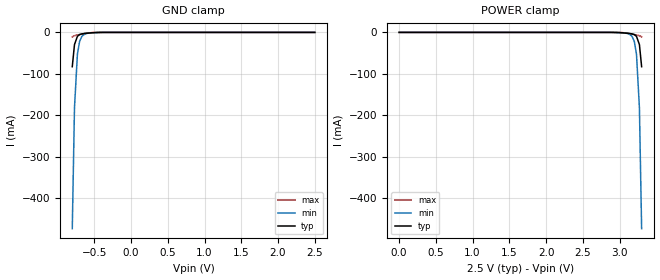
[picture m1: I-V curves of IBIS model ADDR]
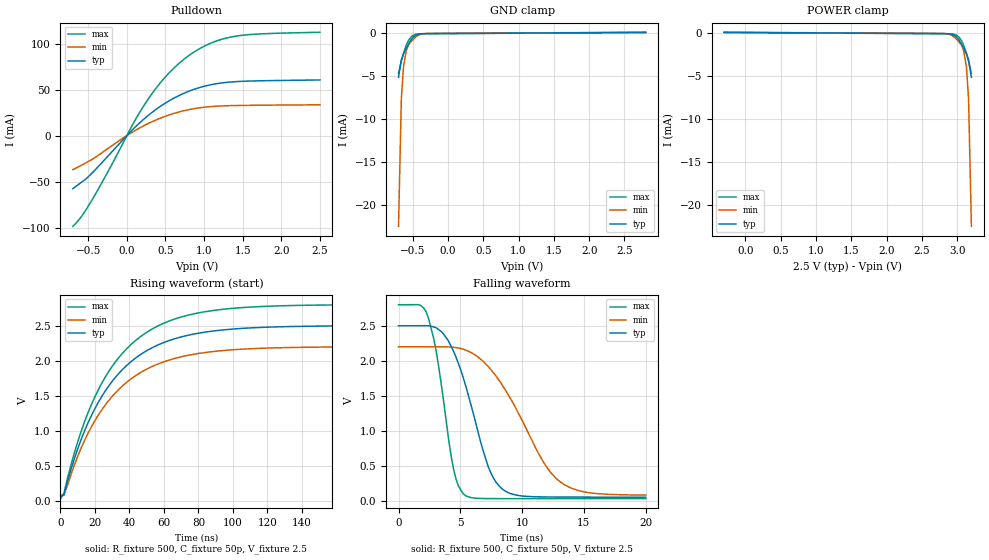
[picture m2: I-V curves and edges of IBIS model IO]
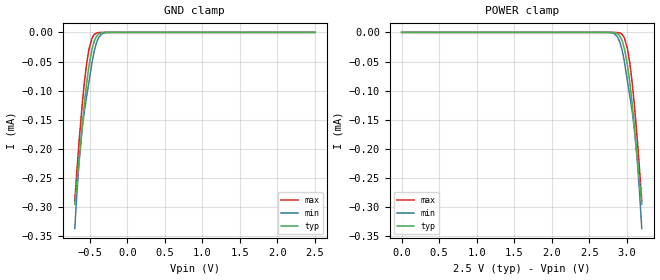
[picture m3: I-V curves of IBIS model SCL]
[IBIS Ver]   3.2
[Comment Char]   |_char
| VDD nom = 2.5v, min = 2.2v, max = 2.8v
[File name]   pca8575_2_5v.ibs
[File Rev]   1
[Date]   Aug 14, 2008 2:49:03 PM
[Source]
Generated by Seshadri Venkataramanan using IBIS Toolkit at NXP Tempe
[Notes]
[Disclaimer]
(C) Copyright 2007 NXP Semiconductors
All rights reserved
NXP Semiconductors (NXP) does not warrant that this model and any other
accompanying information (Model) accurately or fully represents the
operating characteristics and specifications of the semiconductor
products to which the Model relates.  Moreover, the Model is furnished
on an "as is" and with "all faults" basis, and without support or
warranty of any kind.  NXP disclaims all warranties, whether expressed
or implied or statutory, including without limitation all implied
warranties of non-infringement, merchantability and fitness for any
purpose, and those arising from a course of dealing or usage of trade.
NXP does not convey any license under its or any third party's patents,
copyrights or other intellectual property or proprietary rights.
You and your company assume any and all risks and liability arising out
of the application or use of the Model.
In no event shall NXP be liable for any direct, indirect, special,
consequential or incidental damages, however caused, whether in
warranty, contract or tort (including negligence), strict liability or
other legal theory, including, without limitation, for lost profits,
business interruption, or corruption or loss of data or information,
arising out of or in connection with the use of or the inability to use
the Model, even if NXP has been advised of the possibility of such
damages.
NXP provides the Model as a courtesy to our customers. You and your
company shall not distribute, convey, sell, or give the Model to anyone
else without receiving prior written permission from NXP.
NXP reserves the right to make changes without notice to the Model to
improve reliability, function, or design.
Please be aware that your receipt and subsequent use of the Model shall
serve as acceptance of these terms and conditions.  If you do not
accept these terms, return or destroy the Model immediately.
[Copyright]
2008
| SO24 package
[Component]   PCA8575D
Si_location Pin
Timing_location Pin
[Manufacturer]   NXP Semiconductors
[Package]
R_pkg   0.14   0.12   0.18
L_pkg   5.71n   3.95n   7.95n
C_pkg   1.01p   0.72p   1.49p
[Pin] signal_name   model_name   R_pin   L_pin   C_pin
1   INTb   INT_OUT   0.18   6.01n   0.97p
2   AD1   ADDR   0.14   7.94n   1.21p
3   AD2   ADDR   0.16   7.06n   1.32p
4   P00   IO   0.18   6.01n   1.07p
5   P01   IO   0.14   4.98n   0.88p
6   P02   IO   0.13   4.30n   0.80p
7   P03   IO   0.12   3.95n   0.74p
8   P04   IO   0.12   3.95n   0.72p
9   P05   IO   0.13   4.30n   0.76p
10   P06   IO   0.14   4.98n   0.85p
11   P07   IO   0.18   6.01n   0.97p
12   VSS   GND   0.16   7.06n   1.20p
13   P10   IO   0.14   7.95n   1.45p
14   P11   IO   0.14   7.95n   1.49p
15   P12   IO   0.16   7.06n   1.32p
16   P13   IO   0.18   6.01n   1.07p
17   P14   IO   0.14   4.98n   0.88p
18   P15   IO   0.13   4.30n   0.80p
19   P16   IO   0.12   3.95n   0.74p
20   P17   IO   0.12   3.95n   0.72p
21   AD0   ADDR   0.13   4.30n   0.76p
22   SCL   SCL   0.14   4.98n   0.85p
23   SDA   SDAIO   0.18   6.01n   0.97p
24   VDD   POWER   0.16   7.06n   1.20p
| TSSOP24 package
[Component]   PCA8575PW
Si_location Pin
Timing_location Pin
[Manufacturer]   NXP Semiconductors
[Package]
R_pkg   52.70m   31.50m   67.00m
L_pkg   2.19n   1.32n   3.39n
C_pkg   0.48p   0.35p   0.93p
[Pin] signal_name   model_name   R_pin   L_pin   C_pin
1   INTb   INT_OUT   66.40m   2.36n   0.47p
2   AD1   ADDR   66.10m   3.39n   0.57p
3   AD2   ADDR   67.00m   2.94n   0.59p
4   P00   IO   66.40m   2.36n   0.47p
5   P01   IO   47.10m   1.67n   0.40p
6   P02   IO   38.00m   1.44n   0.37p
7   P03   IO   31.50m   1.32n   0.35p
8   P04   IO   31.50m   1.32n   0.35p
9   P05   IO   38.00m   1.44n   0.37p
10   P06   IO   47.10m   1.67n   0.40p
11   P07   IO   66.40m   2.36n   0.47p
12   VSS   GND   67.00m   2.94n   0.59p
13   P10   IO   66.10m   3.39n   0.61p
14   P11   IO   66.20m   3.39n   0.61p
15   P12   IO   67.00m   2.94n   0.59p
16   P13   IO   66.50m   2.36n   0.47p
17   P14   IO   47.10m   1.67n   0.40p
18   P15   IO   38.00m   1.45n   0.37p
19   P16   IO   31.50m   1.32n   0.35p
20   P17   IO   31.50m   1.32n   0.35p
21   AD0   ADDR   38.00m   1.45n   0.37p
22   SCL   SCL   47.10m   1.67n   0.40p
23   SDA   SDAIO   66.50m   2.36n   0.47p
24   VDD   POWER   67.00m   2.94n   0.59p
| SSOP24
[Component]   PCA8575DB
Si_location Pin
Timing_location Pin
[Manufacturer]   NXP Semiconductors
[Package]
R_pkg   54.20m   39.70m   64.80m
L_pkg   2.55n   1.89n   3.58n
C_pkg   0.636p   0.52p   1.05p
[Pin] signal_name   model_name   R_pin   L_pin   C_pin
1   INTb   INT_OUT   63.00m   2.53n   0.58p
2   AD1   ADDR   61.20m   3.56n   0.70p
3   AD2   ADDR   64.80m   3.10n   0.76p
4   P00   IO   63.00m   2.53n   0.60p
5   P01   IO   52.60m   2.17n   0.57p
6   P02   IO   43.90m   2.03n   0.56p
7   P03   IO   39.70m   1.89n   0.54p
8   P04   IO   39.70m   1.89n   0.52p
9   P05   IO   43.90m   2.03n   0.55p
10   P06   IO   52.60m   2.17n   0.56p
11   P07   IO   63.00m   2.53n   0.58p
12   VSS   GND   64.80m   3.10n   0.71p
13   P10   IO   61.20m   3.56n   1.01p
14   P11   IO   61.20m   3.56n   1.05p
15   P12   IO   64.80m   3.10n   0.80p
16   P13   IO   63.00m   2.53n   0.65p
17   P14   IO   52.60m   2.17n   0.59p
18   P15   IO   43.90m   2.03n   0.56p
19   P16   IO   39.70m   1.89n   0.54p
20   P17   IO   39.70m   1.89n   0.53p
21   AD0   ADDR   43.90m   2.03n   0.56p
22   SCL   SCL   52.60m   2.17n   0.57p
23   SDA   SDAIO   63.00m   2.53n   0.60p
24   VDD   POWER   64.80m   3.10n   0.76p
[Define Package Model]  HVQFN24
[Manufacturer]  ST-NXP Wireless
|[Simulated] Chris Hunat
|[Approved] Wayne Nunn, Roger Real
[OEM]  Unknown
[Description]  Full package model
[Number Of Pins]  23
[Pin Numbers]
pin1   | pin1 = lead1
pin2   | pin2 = lead2
pin3   | pin3 = lead3
pin4   | pin4 = lead4
pin5   | pin5 = lead5
pin6   | pin6 = lead6
pin7   | pin7 = lead7
pin8   | pin8 = lead8
pin9   | pin9 = lead9
pin10   | pin10 = lead10
pin11   | pin11 = lead11
pin12   | pin12 = lead12
pin13   | pin13 = lead13
pin14   | pin14 = lead14
pin15   | pin15 = lead15
pin17   | pin17 = lead17
pin18   | pin18 = lead18
pin19   | pin19 = lead19
pin20   | pin20 = lead20
pin21   | pin21 = lead21
pin22   | pin22 = lead22
pin23   | pin23 = lead23
pin24   | pin24 = lead24
[Model Data]
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[End Model Data]
[End Package Model]
[Define Package Model]  DHVQFN24
[Manufacturer]  ST-NXP Wireless
|[Simulated] Chris Hunat
|[Approved] Wayne Nunn, Roger Real
[OEM]  Unknown
[Description]  Full package model
[Number Of Pins]  24
[Pin Numbers]
|Pin Num   Terminal Name
1   | lead1:pin1
2   | lead2:pin2
3   | lead3:pin3
4   | lead4:pin4
5   | lead5:pin5
6   | lead6:pin6
7   | lead7:pin7
8   | lead8:pin8
9   | lead9:pin9
10   | lead10:pin10
11   | lead11:pin11
12   | lead12:pin12
13   | lead13:pin13
14   | lead14:pin14
15   | lead15:pin15
16   | lead16:pin16
17   | lead17:pin17
18   | lead18:pin18
19   | lead19:pin19
20   | lead20:pin20
21   | lead21:pin21
22   | lead22:pin22
23   | lead23:pin23
24   | lead24:pin24
[Model Data]
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[End Model Data]
[End Package Model]
| Models and submodels in the file (5): ADDR (Input), IO (I/O_open_drain), SCL (Input), SDAIO (I/O_open_drain), INT_OUT (Open_drain)
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[Model]   ADDR
Model_type Input
Vinh=1.75
Vinl=0.75
C_comp   0.73p   0.7p   0.76p
[Temperature Range] 27   85   -40
[Voltage Range]   2.5   2.2   2.8
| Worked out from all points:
|   GND clamp passes 1 mA (typ) near -0.54 V on its own axis
[GND Clamp]
-800mV    -82.74mA   -473.3mA   -10.75mA
-770mV    -29.45mA   -181.8mA   -8mA
-730mV    -9.51mA    -52.32mA   -6.198mA
-700mV    -5.302mA   -21.58mA   -5.122mA
-670mV    -3.609mA   -9.611mA   -3.955mA
-630mV    -2.557mA   -3.927mA   -2.533mA
-600mV    -2.04mA    -2.358mA   -1.687mA
-400mV    -48.21uA   -135uA     -7.763uA
2.5V      45.96pA    196.9pA    32.65pA
[POWER Clamp]
0V        45.96pA    196.9pA    32.65pA
2.9V      -48.21uA   -135uA     -7.763uA
3.1V      -2.04mA    -2.358mA   -1.687mA
3.13V     -2.557mA   -3.927mA   -2.533mA
3.17V     -3.609mA   -9.611mA   -3.955mA
3.2V      -5.302mA   -21.58mA   -5.122mA
3.23V     -9.51mA    -52.32mA   -6.198mA
3.27V     -29.45mA   -181.8mA   -8mA
3.3V      -82.74mA   -473.3mA   -10.75mA
[Model]   IO
Model_type I/O_open_drain
Vinh=1.75
Vinl=0.75
Vref=2.5
Vmeas=1.25
Rref=500
Cref=50p
C_comp   6.3p   6.1p   6.5p
[Temperature Range] 27   85   -40
[Voltage Range]   2.5   2.2   2.8
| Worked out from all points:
|   slope of the pulldown table from 0 to 0.375 V, typ, clamps not added: 13.2 ohm
|   GND clamp passes 1 mA (typ) near -0.53 V on its own axis
|   falling waveform, R_fixture 500, C_fixture 50p, V_fixture 2.5: 20-80 % time 2.42ns typ, 3.99ns min, 1.39ns max; typ from 2.5 V to 0.056 V
|   rising waveform, R_fixture 500, C_fixture 50p, V_fixture 2.5: 20-80 % time 34.8ns typ, 34.9ns min, 34.7ns max; typ from 0.055 V to 2.5 V
[Pulldown]
-700mV    -57.71mA   -36.98mA   -98.68mA
-600mV    -51.44mA   -32.7mA    -89.33mA
-470mV    -42.32mA   -26.78mA   -72.62mA
-220mV    -19.92mA   -12.41mA   -35.28mA
80mV      7.081mA    4.274mA    12.86mA
270mV     21.62mA    12.98mA    39.14mA
500mV     35.58mA    21.22mA    64.11mA
750mV     46.61mA    27.43mA    83.97mA
1.05V     54.82mA    31.45mA    99.43mA
1.37V     58.64mA    32.78mA    107.8mA
1.72V     59.78mA    33.18mA    110.8mA
2.5V      60.68mA    33.65mA    112.6mA
[GND Clamp]
-700mV    -5.175mA   -22.41mA   -4.722mA
-660mV    -3.154mA   -7.706mA   -3.345mA
-630mV    -2.474mA   -3.985mA   -2.421mA
-590mV    -1.842mA   -2.07mA    -1.458mA
-560mV    -1.355mA   -1.462mA   -941.6uA
-520mV    -814.4uA   -1.028mA   -497.6uA
-450mV    -303.4uA   -472.4uA   -195.6uA
-380mV    -152.4uA   -185.9uA   -149.5uA
-280mV    -124.3uA   -108.4uA   -141.8uA
2.8V      13.37uA    26.27uA    84.15pA
[POWER Clamp]
-300mV    13.37uA    26.27uA    84.15pA
2.78V     -124.3uA   -108.4uA   -141.8uA
2.88V     -152.4uA   -185.9uA   -149.5uA
2.95V     -303.4uA   -472.4uA   -195.6uA
3.02V     -814.4uA   -1.028mA   -497.6uA
3.06V     -1.355mA   -1.462mA   -941.6uA
3.09V     -1.842mA   -2.07mA    -1.458mA
3.13V     -2.474mA   -3.985mA   -2.421mA
3.16V     -3.154mA   -7.706mA   -3.345mA
3.2V      -5.175mA   -22.41mA   -4.722mA
[Falling Waveform]
R_fixture=500
C_fixture=50p
V_fixture=2.5
V_fixture_min=2.2
V_fixture_max=2.8
0s        2.5V       2.2V       2.8V
1.818ns   2.501V     2.2V       2.787V
2.424ns   2.5V       2.201V     2.608V
3.03ns    2.473V     2.201V     2.155V
4.444ns   2.141V     2.193V     463.6mV
5.253ns   1.751V     2.165V     101.4mV
7.273ns   485mV      1.917V     35.58mV
8.485ns   160.6mV    1.629V     34.55mV
13.13ns   57.19mV    268.7mV    34.02mV
20ns      55.56mV    85.37mV    34.01mV
[Rising Waveform]
R_fixture=500
C_fixture=50p
V_fixture=2.5
V_fixture_min=2.2
V_fixture_max=2.8
0s        55.5mV     81.08mV    34.01mV
2.02ns    90.22mV    82.73mV    111.6mV
8.081ns   604.3mV    514.3mV    688.4mV
14.14ns   1.01V      873.6mV    1.142V
24.24ns   1.503V     1.311V     1.692V
36.36ns   1.885V     1.65V      2.118V
52.53ns   2.177V     1.911V     2.443V
70.71ns   2.344V     2.06V      2.628V
96.97ns   2.445V     2.151V     2.74V
200ns     2.499V     2.199V     2.799V
[Ramp]
R_load=500
dV/dt_r   1.467E+0/9.967E-10   1.441E+0/1.134E-9   1.486E+0/8.761E-10
dV/dt_f   1.467E+0/7.542E-10   1.439E+0/1.579E-9   1.486E+0/3.233E-10
|[End   IO
[Model]   SCL
Model_type Input
Vinh=1.75
Vinl=0.75
C_comp   2.1p   1.9p   2.3p
[Temperature Range] 27   85   -40
[Voltage Range]   2.5   2.2   2.8
[GND Clamp]
-700mV    -295uA     -337uA     -289.5uA
-670mV    -255uA     -273.2uA   -234.2uA
-640mV    -215uA     -219.5uA   -182.9uA
-600mV    -158.8uA   -164.3uA   -122uA
-570mV    -119.6uA   -133.4uA   -83.31uA
-540mV    -85.29uA   -108.2uA   -51.83uA
-510mV    -56.75uA   -84.45uA   -28.37uA
-470mV    -28.59uA   -51.28uA   -9.682uA
-440mV    -14.75uA   -31.48uA   -3.492uA
-380mV    -2.609uA   -8.444uA   -299.4nA
-340mV    -638.4nA   -2.69uA    -49.05nA
2.5V      6.036pA    19.25pA    5.008pA
[POWER Clamp]
0V        6.036pA    19.25pA    5.008pA
2.84V     -638.4nA   -2.69uA    -49.05nA
2.88V     -2.609uA   -8.444uA   -299.4nA
2.94V     -14.75uA   -31.48uA   -3.492uA
2.97V     -28.59uA   -51.28uA   -9.682uA
3.01V     -56.75uA   -84.45uA   -28.37uA
3.04V     -85.29uA   -108.2uA   -51.83uA
3.07V     -119.6uA   -133.4uA   -83.31uA
3.1V      -158.8uA   -164.3uA   -122uA
3.14V     -215uA     -219.5uA   -182.9uA
3.17V     -255uA     -273.2uA   -234.2uA
3.2V      -295uA     -337uA     -289.5uA
